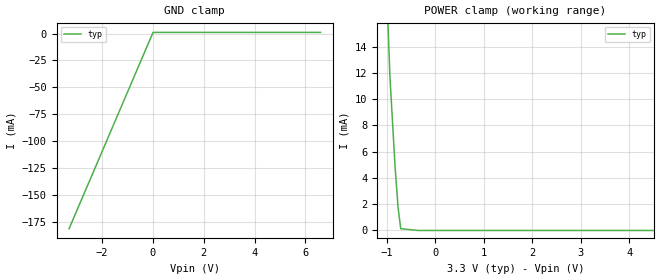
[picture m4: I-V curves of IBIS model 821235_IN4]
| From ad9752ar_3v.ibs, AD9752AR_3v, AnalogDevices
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| COPYRIGHT(C) MENTOR GRAPHICS CORPORATION 2002 ALL
| RIGHTS RESERVED. THIS WORK CONTAINS PROPRIETARY
| INFORMATION WHICH IS THE PROPERTY OF MENTOR GRAPHICS
| CORPORATION OR ITS LICENSORS. USE OF THESE MATERIALS
| IS SUBJECT TO THE TERMS BELOW.
| USE: MENTOR GRAPHICS HAS LICENSED IBIS MODELS TO
| SPECIFIC INTEGRATED CIRCUIT SUPPLIERS ("IC VENDORS")
| FOR USE AND DISTRIBUTION AS FOLLOWS: EACH IC VENDOR
| MAY USE IBIS MODELS, AND DISTRIBUTE THEM TO IC VENDOR'S
| CUSTOMERS TO USE, SOLELY FOR DEVELOPING PRINTED
| CIRCUIT BOARD DESIGNS. NO OTHER USE OR DISTRIBUTION
| OF THESE MATERIALS IS PERMITTED.
| Model Application Version 1.89 2/18/99.
[Model] 821235_IN4
Model_type Input
Vinl = 900.0mV
Vinh = 2.100V
C_comp 5.000pF NA NA
| variable typ   min   max
[Voltage Range] 3.300V NA NA
[GND Clamp Reference] 0.000V NA NA
[POWER Clamp Reference] 3.300V NA NA
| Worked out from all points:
|   POWER clamp passes 1 mA (typ) near -0.74 V on its own axis
[GND Clamp]
-3.3V     -181.3mA   NA         NA
5.311mV   1.099mA    NA         NA
6.6V      1.099mA    NA         NA
[POWER Clamp]
-3.3V     332.9mA    NA         NA
-1.058V   23.88mA    NA         NA
-936.8mV  11.71mA    NA         NA
-830.5mV  4.849mA    NA         NA
-769.6mV  1.779mA    NA         NA
-713.8mV  137.2uA    NA         NA
-356.9mV  0A         NA         NA
6.6V      0A         NA         NA
